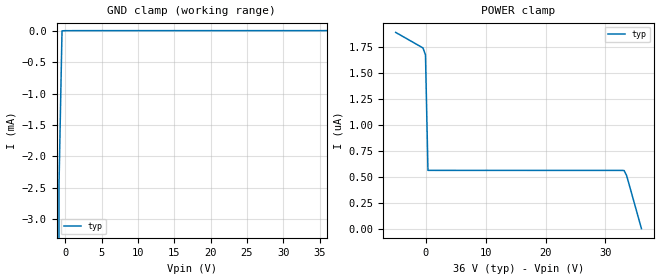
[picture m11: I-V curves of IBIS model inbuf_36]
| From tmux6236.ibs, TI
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| inbuf_36
[Model]   inbuf_36
Model_type   Input
Vinl = 0.8
Vinh = 1.3
|   typ   min   max
C_comp   4.014581e-13   NA   NA
[Voltage Range]   36   NA   NA
[Temperature Range]   27   NA   NA
[Power Clamp Reference]   36   NA   NA
[GND Clamp Reference]   0   NA   NA
[GND Clamp]
|   Voltage   I(typ)   I(min)   I(max)
-5V       -1.213A    NA         NA
-1.273V   -74.84mA   NA         NA
-858.6mV  -2.444mA   NA         NA
-444.4mV  -3.239uA   NA         NA
36V       1.588uA    NA         NA
[POWER Clamp]
|   Voltage   I(typ)   I(min)   I(max)
-5V       1.887uA    NA         NA
-444.4mV  1.737uA    NA         NA
-30.3mV   1.67uA     NA         NA
383.8mV   560.2nA    NA         NA
33.1V     558.8nA    NA         NA
33.52V    511.5nA    NA         NA
36V       -195.5pA   NA         NA
